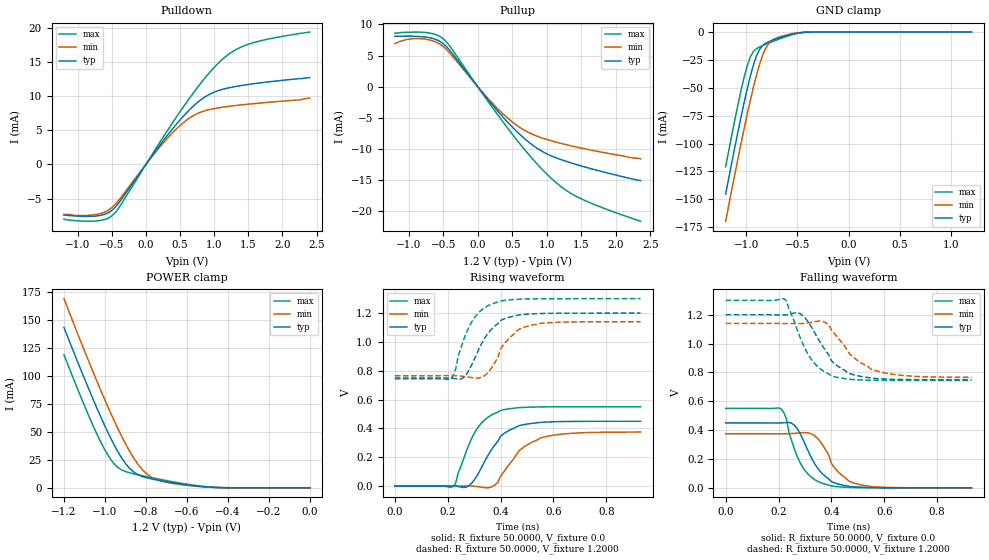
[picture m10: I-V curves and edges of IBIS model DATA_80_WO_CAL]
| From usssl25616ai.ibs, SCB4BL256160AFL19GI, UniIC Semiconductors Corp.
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|   Model DATA_80_WO_CAL
[Model]  DATA_80_WO_CAL
Model_type I/O
Polarity   Non-Inverting
Enable   Active-High
Vinl =   0.3800V
Vinh =   0.8200V
Vmeas =  0.6000V
Cref =   5.0000pF
Rref =   50.0000
Vref =   0.6000V
C_comp   1.7430pF   1.7110pF   1.7640pF
[Temperature Range]   25.0000   85.0000   -40.0000
[Voltage Range]   1.2000V   1.1400V   1.3000V
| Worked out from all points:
|   slope of the pulldown table from 0 to 0.18 V, typ, clamps not added: 72.3 ohm
|   slope of the pullup table from 0 to 0.18 V, typ, clamps not added: 72.5 ohm
|   GND clamp passes 1 mA (typ) near -0.50 V on its own axis
|   POWER clamp passes 1 mA (typ) near -0.51 V on its own axis
|   rising waveform, R_fixture 50.0000, V_fixture 0.0: 20-80 % time 93.1ps typ, 111ps min, 85.6ps max; typ from 0 V to 0.45 V
|   rising waveform, R_fixture 50.0000, V_fixture 1.2000: 20-80 % time 87.8ps typ, 83.6ps min, 75.5ps max; typ from 0.75 V to 1.2 V
|   falling waveform, R_fixture 50.0000, V_fixture 0.0: 20-80 % time 84.5ps typ, 83ps min, 71ps max; typ from 0.45 V to 0 V
|   falling waveform, R_fixture 50.0000, V_fixture 1.2000: 20-80 % time 102ps typ, 124ps min, 87.9ps max; typ from 1.2 V to 0.75 V
[Pulldown]
|Voltage   I(typ)   I(min)   I(max)
-1.2V     -7.4mA     -7.3mA     -8mA
-720mV    -7.53mA    -7.3mA     -8.257mA
-480mV    -6.557mA   -6.151mA   -7.359mA
-360mV    -5.125mA   -4.751mA   -5.782mA
200mV     2.759mA    2.501mA    3.175mA
520mV     6.727mA    5.862mA    7.998mA
680mV     8.39mA     7.046mA    10.24mA
840mV     9.703mA    7.766mA    12.33mA
1.2V      11.16mA    8.471mA    16.02mA
1.4V      11.54mA    8.704mA    17.18mA
1.6V      11.83mA    8.903mA    17.87mA
2.4V      12.7mA     9.7mA      19.35mA
[Pullup]
|Voltage   I(typ)   I(min)   I(max)
-1.2V     8.1mA      6.9mA      8.6mA
-880mV    8.08mA     7.73mA     8.76mA
-680mV    7.819mA    7.448mA    8.569mA
-520mV    7.078mA    6.632mA    7.875mA
-400mV    5.766mA    5.348mA    6.459mA
120mV     -1.673mA   -1.541mA   -1.9mA
440mV     -5.77mA    -5.1mA     -6.744mA
760mV     -9.09mA    -7.482mA   -11.15mA
1.08V     -11.18mA   -8.733mA   -14.87mA
1.28V     -11.99mA   -9.309mA   -16.64mA
1.48V     -12.67mA   -9.815mA   -17.91mA
2.36V     -15.1mA    -11.6mA    -21.62mA
[GND_clamp]
|Voltage   I(typ)   I(min)   I(max)
-1.2V     -145.3mA   -169.7mA   -120.8mA
-1.11V    -103.1mA   -127.3mA   -78.51mA
-1.05V    -76.2mA    -100.1mA   -52.43mA
-990mV    -51.2mA    -74mA      -30.39mA
-960mV    -39.9mA    -61.63mA   -22.48mA
-900mV    -21.67mA   -39mA      -15mA
-870mV    -15.78mA   -29.25mA   -13.45mA
-810mV    -10.04mA   -14.72mA   -11.07mA
-750mV    -7.557mA   -7.71mA    -8.865mA
-600mV    -3.111mA   -2.463mA   -3.804mA
-420mV    -215.4uA   -156.1uA   -235uA
1.2V      1.597nA    5.589nA    1.463nA
[POWER_clamp]
|Voltage   I(typ)   I(min)   I(max)
-1.2V     143mA      168.8mA    118.7mA
-1.06V    79.88mA    104.3mA    56.26mA
-1.02V    63.08mA    86.79mA    40.63mA
-980mV    47.32mA    69.97mA    27.48mA
-940mV    33.2mA     54.05mA    18.67mA
-880mV    17.43mA    32.78mA    13.45mA
-840mV    11.87mA    21.34mA    11.69mA
-800mV    9.133mA    13.1mA     10.12mA
-720mV    6.135mA    5.731mA    7.166mA
-560mV    1.838mA    1.456mA    2.161mA
-420mV    156.9uA    132.7uA    153uA
0V        1.597nA    1.927nA    2.16nA
[Ramp]
| variable   typ   min   max
dV/dt_r  0.2701/95.9095p   0.2251/0.1128n   0.3305/79.6325p
dV/dt_f  0.2703/0.1038n   0.2243/0.1251n   0.3332/81.7811p
R_load = 50.0000
[Rising Waveform]
R_fixture= 50.0000
V_fixture= 0.0
V_fixture_min= 0.0
V_fixture_max= 0.0
|time   V(typ)   V(min)   V(max)
0s        0V         0V         0V
220ps     1.302mV    184.3uV    -3.005mV
230ps     1.356mV    333.6uV    20.35mV
270ps     -7.188mV   1.346mV    239.7mV
310ps     69.87mV    -1.76mV    395.1mV
370ps     264.3mV    -1.272mV   497.7mV
400ps     346.6mV    69.12mV    524.9mV
470ps     419.3mV    245.5mV    544.6mV
550ps     442.3mV    333.8mV    549.5mV
930ps     450.1mV    375.1mV    550.8mV
[Rising Waveform]
R_fixture= 50.0000
V_fixture= 1.2000
V_fixture_min= 1.1400
V_fixture_max= 1.3000
|time   V(typ)   V(min)   V(max)
0s        749.5mV    765.7mV    744.6mV
210ps     748.3mV    766.3mV    740.6mV
230ps     745.3mV    765.9mV    809.4mV
260ps     752.1mV    760.9mV    1.012V
300ps     876.7mV    750.3mV    1.165V
350ps     1.053V     782.4mV    1.248V
400ps     1.148V     951.4mV    1.283V
470ps     1.187V     1.087V     1.296V
550ps     1.197V     1.128V     1.299V
930ps     1.2V       1.14V      1.3V
[Falling Waveform]
R_fixture= 50.0000
V_fixture= 0.0
V_fixture_min= 0.0
V_fixture_max= 0.0
|time   V(typ)   V(min)   V(max)
0s        450.1mV    375.3mV    550.8mV
210ps     450.5mV    374.8mV    547.6mV
230ps     452.6mV    374.9mV    478.1mV
250ps     447.6mV    376.4mV    324.7mV
290ps     344.9mV    381.9mV    148.1mV
330ps     188.6mV    369.1mV    65.62mV
370ps     90.71mV    288.3mV    28.97mV
420ps     29.49mV    122.4mV    8.486mV
490ps     6.533mV    30.45mV    1.649mV
930ps     748nV      6.721uV    0V
[Falling Waveform]
R_fixture= 50.0000
V_fixture= 1.2000
V_fixture_min= 1.1400
V_fixture_max= 1.3000
|time   V(typ)   V(min)   V(max)
0s        1.2V       1.14V      1.3V
220ps     1.199V     1.139V     1.312V
230ps     1.199V     1.139V     1.297V
290ps     1.197V     1.139V     1.006V
340ps     1.065V     1.153V     855.4mV
380ps     947.4mV    1.143V     798.9mV
400ps     882.1mV    1.095V     776.3mV
470ps     791.7mV    926.6mV    752mV
560ps     759.1mV    817.3mV    745.8mV
930ps     749.5mV    766.1mV    744.6mV
